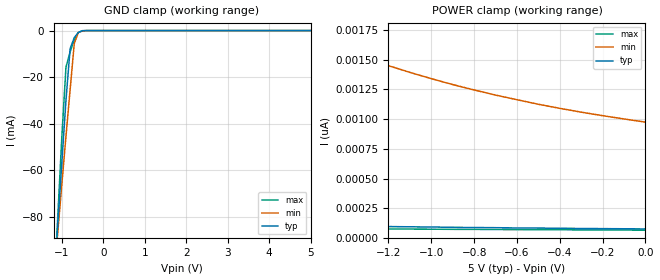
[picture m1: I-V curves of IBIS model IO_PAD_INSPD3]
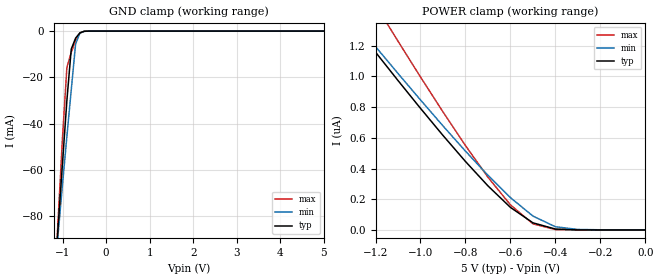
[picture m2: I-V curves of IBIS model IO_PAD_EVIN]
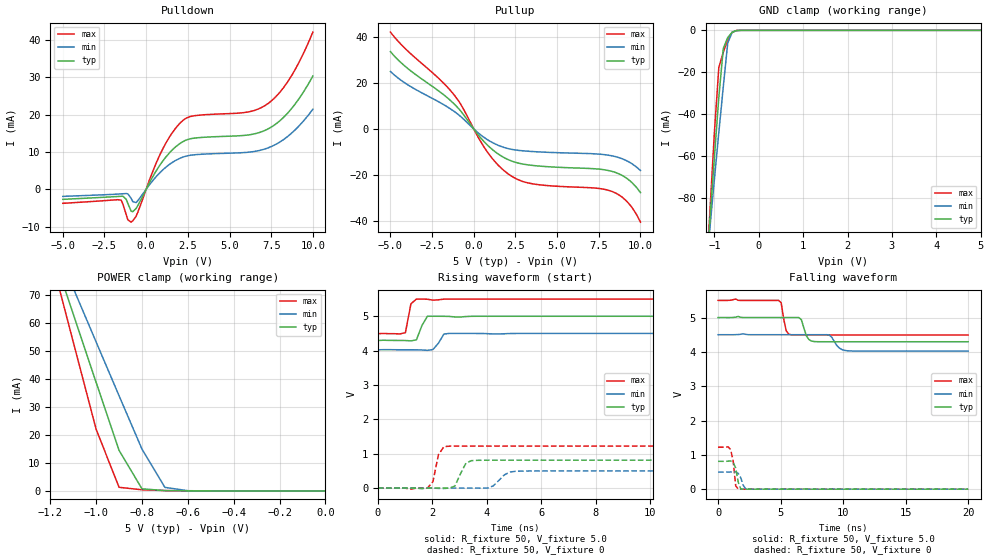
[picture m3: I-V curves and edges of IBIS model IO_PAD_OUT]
[IBIS Ver]   3.2
[Comment Char]   |_char
[File name]   r8804ce_50v.ibs
[File Rev]   1.0
[Date]   2018/09/06 15:44:38
[Source]
[Notes]
[Disclaimer]
This information is for modeling purposes only, and is not guaranteed.
Property of SEIKO EPSON Corp.,
unauthorized reproduction and/or distribution is strictly prohibited.
[Copyright]
Copyright 2018, SEIKO EPSON Corp.
[Component]   r8804ce50v
Si_location Pin
Timing_location Pin
[Manufacturer]   SEIKO EPSON Corp.
| RA/RX-8804CE
[Package]
R_pkg   267m   NA   NA
L_pkg   2.8nH   NA   NA
C_pkg   0.70pF   NA   NA
[Pin] signal_name   model_name
1   FOE   IO_PAD_INSPD3
2   Vdd   POWER
3   EVIN   IO_PAD_EVIN
4   FOUT   IO_PAD_OUT
5   SCL   IO_PAD_INSPD2
6   SOUT   IO_PAD_DIO
7   SDA   IO_PAD_DIO_SMT
8   Vpp   POWER
9   GND   GND
10   /INT   IO_PAD_XINT
| Models and submodels in the file (7): IO_PAD_INSPD3 (Input), IO_PAD_EVIN (Input), IO_PAD_OUT (3-state), IO_PAD_INSPD2 (Input), IO_PAD_DIO (I/O), IO_PAD_DIO_SMT (I/O_open_drain), IO_PAD_XINT (Open_drain)
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[Model]   IO_PAD_INSPD3
Model_type Input
Enable Active-High
Polarity Non-Inverting
Vinh=4.4
Vinl=0.9
C_comp   2.5p   2.0p   3.0p
[Temperature Range] 25   105   -40
[Voltage Range]   5.0   4.5   5.5
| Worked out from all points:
|   GND clamp passes 1 mA (typ) near -0.61 V on its own axis
[GND Clamp]
-5V       -1.197A    -967.6mA   -1.498A
-1.2V     -111.6mA   -108.8mA   -116mA
-1.1V     -84.12mA   -87.28mA   -80.81mA
-1V       -56.82mA   -66.06mA   -45.85mA
-900mV    -29.96mA   -45.45mA   -15.68mA
-800mV    -7.806mA   -25.48mA   -9.236mA
-700mV    -3.032mA   -5.589mA   -3.961mA
-600mV    -756.3uA   -818.5uA   -830.7uA
-500mV    -74.57uA   -117.4uA   -45.32uA
-400mV    -4.08uA    -12.66uA   -921.8nA
5V        75.72pA    1.125nA    59.46pA
[POWER Clamp]
-5V       290.8pA    9.048nA    108.9pA
-4.2V     223.3pA    6.202nA    100.3pA
-3.4V     172.3pA    4.166nA    93.22pA
-2.7V     139.8pA    2.92nA     87.54pA
-1.7V     107.5pA    1.797nA    78.9pA
-1.6V     105.5pA    1.718nA    78.22pA
-1.4V     100.3pA    1.575nA    76.4pA
-1.2V     95.72pA    1.45nA     74.81pA
-1V       92.09pA    1.34nA     73.67pA
-800mV    87.54pA    1.245nA    72.08pA
-400mV    81.51pA    1.09nA     69.35pA
0V        75.72pA    974.4pA    65.26pA
[Model]   IO_PAD_EVIN
Model_type Input
Enable Active-High
Polarity Non-Inverting
Vinh=4.4
Vinl=0.9
C_comp   2.5p   2.0p   3.0p
[Temperature Range] 25   105   -40
[Voltage Range]   5.0   4.5   5.5
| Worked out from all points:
|   GND clamp passes 1 mA (typ) near -0.61 V on its own axis
[GND Clamp]
-5V       -1.197A    -967.6mA   -1.498A
-1.2V     -111.6mA   -108.8mA   -116mA
-1.1V     -84.12mA   -87.28mA   -80.81mA
-1V       -56.82mA   -66.06mA   -45.85mA
-900mV    -29.96mA   -45.45mA   -15.68mA
-800mV    -7.806mA   -25.48mA   -9.236mA
-700mV    -3.032mA   -5.589mA   -3.961mA
-600mV    -756.3uA   -818.5uA   -830.7uA
-500mV    -74.57uA   -117.4uA   -45.32uA
-400mV    -4.08uA    -12.66uA   -921.8nA
5V        75.72pA    90.36nA    58.55pA
[POWER Clamp]
-5V       9.282uA    8.698uA    11.73uA
-1.3V     1.346uA    1.371uA    1.708uA
-1.2V     1.158uA    1.194uA    1.467uA
-1.1V     973.3nA    1.019uA    1.23uA
-900mV    615.7nA    677.8nA    768.8nA
-800mV    446nA      513.3nA    549.4nA
-700mV    287nA      355.8nA    343.3nA
-600mV    146.9nA    210.6nA    163.3nA
-500mV    46.44nA    90.36nA    40.09nA
-400mV    6.011nA    20.89nA    2.674nA
-300mV    415.5pA    3.237nA    124.6pA
0V        75.72pA    974.2pA    65.26pA
[Model]   IO_PAD_OUT
Model_type 3-state
Enable Active-High
Polarity Non-Inverting
Vmeas=2.50
C_comp   2.5p   2.0p   3.0p
[Temperature Range] 25   105   -40
[Voltage Range]   5.0   4.5   5.5
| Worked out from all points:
|   slope of the pulldown table from 0 to 0.75 V, typ, clamps not added: 126 ohm
|   slope of the pullup table from 0 to 0.75 V, typ, clamps not added: 116 ohm
|   GND clamp passes 1 mA (typ) near -0.61 V on its own axis
|   POWER clamp passes 1 mA (typ) near -0.80 V on its own axis
|   falling waveform, R_fixture 50, V_fixture 5.0: 20-80 % time 392ps typ, 551ps min, 302ps max; typ from 5 V to 4.29 V
|   falling waveform, R_fixture 50, V_fixture 0: 20-80 % time 287ps typ, 326ps min, 256ps max; typ from 0.812 V to 0 V
|   rising waveform, R_fixture 50, V_fixture 5.0: 20-80 % time 239ps typ, 249ps min, 146ps max; typ from 4.29 V to 5 V
|   rising waveform, R_fixture 50, V_fixture 0: 20-80 % time 296ps typ, 396ps min, 195ps max; typ from 0 V to 0.812 V
[Pullup]
-5V       33.52mA    24.92mA    42mA
-3.9V     25.87mA    18.88mA    33.39mA
-2.1V     16.45mA    11.75mA    21.92mA
-1.2V     11.01mA    7.73mA     14.97mA
-800mV    7.926mA    5.5mA      10.92mA
800mV     -6.847mA   -4.548mA   -9.793mA
2V        -13.08mA   -8.393mA   -19.13mA
2.7V      -14.84mA   -9.282mA   -22.1mA
3.5V      -15.78mA   -9.765mA   -23.74mA
8.3V      -18.4mA    -11.66mA   -27.12mA
9.2V      -21.51mA   -13.88mA   -31.53mA
10V       -27.61mA   -18.03mA   -40.4mA
[Pulldown]
-5V       -2.695mA   -1.899mA   -3.76mA
-1.5V     -1.871mA   -1.232mA   -2.909mA
-1.1V     -3.756mA   -1.223mA   -8.145mA
-900mV    -5.868mA   -2.416mA   -8.805mA
-600mV    -5.116mA   -3.564mA   -7.202mA
900mV     6.952mA    4.772mA    9.936mA
2V        12.16mA    8.239mA    17.55mA
2.7V      13.56mA    9.131mA    19.52mA
6.1V      14.53mA    9.907mA    20.68mA
7.3V      16.12mA    11.06mA    22.91mA
8.6V      20.95mA    14.55mA    29.52mA
10V       30.3mA     21.42mA    42.06mA
[GND Clamp]
-5V       -1.289A    -1.043A    -1.612A
-1.2V     -119.5mA   -117.1mA   -123.7mA
-1.1V     -89.88mA   -93.83mA   -85.77mA
-1V       -60.41mA   -70.86mA   -48.66mA
-900mV    -31.76mA   -48.51mA   -17.63mA
-800mV    -8.707mA   -26.99mA   -10.46mA
-700mV    -3.454mA   -6.077mA   -4.512mA
-600mV    -868.8uA   -933.9uA   -956.3uA
-500mV    -86.23uA   -135.8uA   -52.66uA
-400mV    -4.725uA   -14.7uA    -1.074uA
5V        56.39pA    6.299uA    31.72pA
[POWER Clamp]
-5V       1.033A     837.7mA    1.291A
-1.2V     87.98mA    92.05mA    84.88mA
-1.1V     63.38mA    72.67mA    53.4mA
-1V       38.87mA    53.34mA    22.09mA
-900mV    14.53mA    34.09mA    1.297mA
-800mV    753.7uA    14.98mA    407.8uA
-700mV    112.9uA    1.273mA    132.2uA
-600mV    21.58uA    77.12uA    21.07uA
0V        56.39pA    1.099nA    41.15pA
[Falling Waveform]
R_fixture=50
V_fixture=5.0
V_fixture_min=4.5
V_fixture_max=5.5
0s        5V         4.5V       5.5V
4.848ns   5V         4.5V       5.501V
5.051ns   5V         4.5V       5.43V
5.455ns   5V         4.5V       4.616V
5.859ns   5V         4.5V       4.496V
6.667ns   4.937V     4.5V       4.492V
7.071ns   4.463V     4.5V       4.492V
7.677ns   4.301V     4.5V       4.492V
10.3ns    4.295V     4.034V     4.492V
20ns      4.295V     4.024V     4.492V
[Falling Waveform]
R_fixture=50
V_fixture=0
V_fixture_min=0
V_fixture_max=0
0s        811.5mV    498.6mV    1.223V
808.1ps   816.3mV    497.6mV    1.235V
1.01ns    822.5mV    501.8mV    1.153V
1.212ns   779.5mV    507.5mV    819.8mV
1.414ns   614.1mV    501.6mV    95.55mV
1.616ns   204mV      457.8mV    623.9uV
1.818ns   4.363mV    332.8mV    41.8uV
2.02ns    257.6uV    108.5mV    -2.499uV
2.222ns   23.07uV    4.36mV     3.656uV
20ns      556.5nV    0V         -1.418uV
[Rising Waveform]
R_fixture=50
V_fixture=5.0
V_fixture_min=4.5
V_fixture_max=5.5
0s        4.295V     4.024V     4.492V
1.01ns    4.294V     4.024V     4.521V
1.212ns   4.283V     4.024V     5.36V
1.414ns   4.313V     4.024V     5.5V
1.616ns   4.728V     4.019V     5.5V
1.818ns   5V         4.008V     5.495V
2.02ns    5V         4.032V     5.468V
2.424ns   4.999V     4.483V     5.498V
2.626ns   4.995V     4.5V       5.5V
20ns      5V         4.5V       5.5V
[Rising Waveform]
R_fixture=50
V_fixture=0
V_fixture_min=0
V_fixture_max=0
0s        0V         0V         0V
1.818ns   -561.5uV   217.9uV    -1.922mV
2.02ns    81.52uV    -1.95mV    186.2mV
2.222ns   65.86uV    -8.313mV   969.1mV
2.626ns   -2.894mV   -6.729uV   1.219V
2.828ns   60.94mV    -17.14uV   1.221V
3.232ns   725.7mV    87.46uV    1.222V
3.636ns   807.7mV    -780.7uV   1.223V
5.051ns   811.5mV    488.3mV    1.223V
20ns      811.5mV    498.6mV    1.223V
[Ramp]
R_load=50
dV/dt_r   4.869E-1/2.571E-10   2.992E-1/3.755E-10   7.336E-1/1.905E-10
dV/dt_f   4.228E-1/3.595E-10   2.856E-1/5.438E-10   6.049E-1/2.541E-10
|[End   IO_PAD_OUT
